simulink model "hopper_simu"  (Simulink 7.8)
settings: Solver=ode1  StartTime=0.0  StopTime=10.0  FixedStep=1e-4  MaxStep=0.01  RelTol=1e-3
undefined symbols (not defined in the file or in its folder): MP

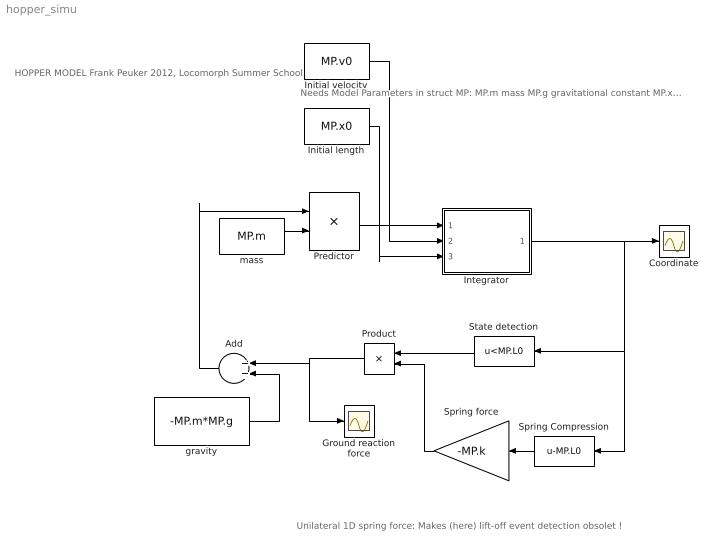
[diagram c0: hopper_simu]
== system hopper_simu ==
  note: Unilateral 1D spring force: Makes (here) lift-off event detection obsolet !
  note: Needs Model Parameters in struct MP: MP.m mass MP.g gravitational constant MP.x0 initial position MP.v0 initial speed MP.L0 rest leg length (e.g. in standing) MP.k stiffness of spring
  note: HOPPER MODEL Frank Peuker 2012, Locomorph Summer School
  Add : Sum
  Coordinate : Scope
  Ground reaction force : Scope
  Initial length : Constant  Value=MP.x0
  Initial velocity : Constant  Value=MP.v0
  Integrator : Subsystem
  Predictor : Product  Inputs=*/
  Product : Product
  Spring Compression : Fcn  Expr=u-MP.L0
  Spring force : Gain  Gain=-MP.k
  State detection : Fcn  Expr=u<MP.L0
  gravity : Constant  Value=-MP.m*MP.g
  mass : Constant  Value=MP.m
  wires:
  Initial velocity/1 -> Integrator/2(v_init)
  Initial length/1 -> Integrator/3(L_init)
  Predictor/1 -> Integrator/1(a)
  mass/1 -> Predictor/2
  Integrator/1(L) -> State detection/1, Spring Compression/1, Coordinate/1
  Add/1 -> Predictor/1
  gravity/1 -> Add/2
  State detection/1 -> Product/1
  Spring force/1 -> Product/2
  Product/1 -> Add/1, Ground reaction force/1
  Spring Compression/1 -> Spring force/1

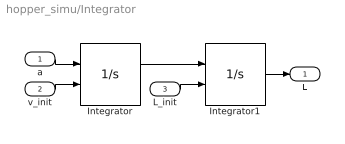
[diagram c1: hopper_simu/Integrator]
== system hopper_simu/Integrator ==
  a : Inport
  v_init : Inport  Port=2
  L_init : Inport  Port=3
  Integrator : Integrator  InitialConditionSource=external
  Integrator1 : Integrator  InitialConditionSource=external
  L : Outport
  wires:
  Integrator/1 -> Integrator1/1
  a/1 -> Integrator/1
  Integrator1/1 -> L/1
  v_init/1 -> Integrator/2
  L_init/1 -> Integrator1/2
